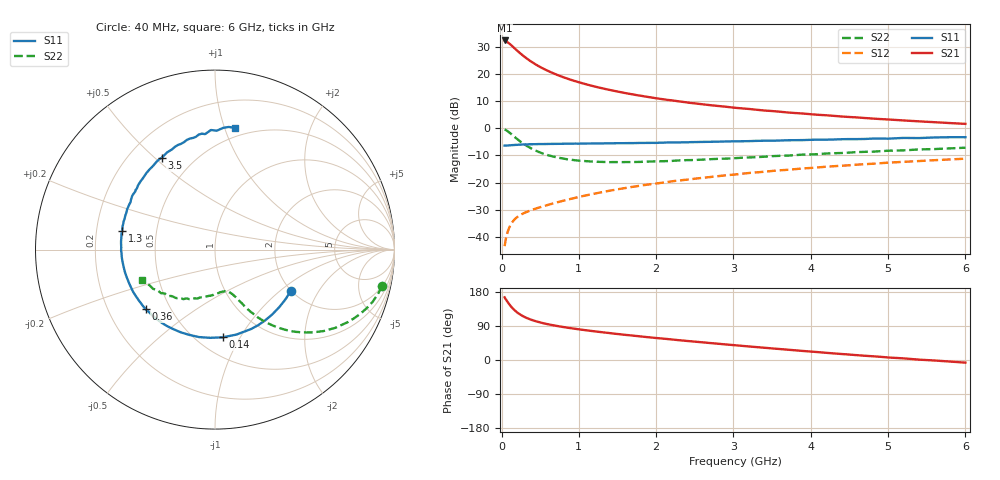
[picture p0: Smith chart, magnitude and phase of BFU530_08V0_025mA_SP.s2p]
! Filename:  P:\Prog\Test\Noise\ATS_data\Testdata_Net\03 Spar\BFU530_APG2013_40_A05_08p0V_025mA_SP_CM01_D.s2p
! Date/Time: Fri 26/Apr/2013 13:03:13
! BFU530_APG2013_40_A05_08p0V_1to25mA_SP_CM01_Bias8_R.s2p
! MDIF S-parameter v. bias file
! BFU530_APG2013_40_A05_08p0V_1to25mA_SP_CM01
! Date/time Wed Apr 24 16:58:28 2013
! VAR V_out= 7.1810
! VAR I_out= 25.0000
! VAR V_in= 0.8207
! VAR I_in= 0.2699
! Device data file deembeded for feedlines and parallel
! Original file: \03 Spar\BFU530_APG2013_40_A05_08p0V_025mA_SP_CM01_R.s2p
! Feed-files: PR047V01_250413_Feed1.s2p, PR047V01_250413_Feed2.s2p
! Parallel-file: PR047V01_250413_Par.s2p
# MHz S MA R 50
!  Freq-MHz  S11-mag  S11-arg  S21-mag  S21-arg  S12-mag  S12-arg  S22-mag  S22-arg
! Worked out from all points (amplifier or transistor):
!   98 points, 40 MHz to 6 GHz, reference 50 ohm
!   highest |S21| = 32.5 dB at 40 MHz (marker M1)
!   |S21| within 3 dB of that: start of sweep to 173.1 MHz
!   unconditionally stable (mu >= 1): 1.194 GHz to 3.436 GHz
!   at 300 MHz: K = 0.52, MSG = 28.8 dB, |S12| = -31.2 dB
!   at 1.6 GHz: K = 1.04, MAG = 16.3 dB, |S12| = -22.1 dB
!   at 6 GHz: K = 0.86, MSG = 6.4 dB, |S12| = -11.2 dB
!   S11 on the Smith chart (normalised r, x): 40 MHz: 2.00, -1.19; 140 MHz: 0.66, -0.85; 360 MHz: 0.36, -0.33; 1.3 GHz: 0.31, +0.09; 3.5 GHz: 0.33, +0.53; 6 GHz: 0.42, +1.08
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40  0.4813 -28.4  42.16 165.4  0.006663 79.8  0.9537 -12.3
50  0.4805 -35.3  41.71 161.6  0.008114 77.7  0.9405 -15.3
90  0.4849 -60.1  37.92 149.8  0.01349 69.5  0.8646 -26.2
120  0.4883 -75.9  35.01 141.8  0.01675 64.6  0.7991 -33.1
140  0.4906 -85.0  33.01 137.2  0.01855 62.0  0.756 -36.9
180  0.4954 -100.3  29.23 129.4  0.02158 58.1  0.676 -43.1
200  0.4962 -106.6  27.53 126.0  0.02279 56.6  0.6399 -45.7
240  0.5002 -117.4  24.55 120.2  0.02491 54.7  0.5769 -49.9
300  0.5052 -129.9  20.92 113.4  0.02759 53.2  0.5024 -54.5
360  0.5095 -139.3  18.1 108.1  0.02992 52.7  0.4461 -57.8
460  0.5119 -150.8  14.68 101.4  0.03356 53.3  0.379 -61.3
600  0.5152 -162.0  11.57 94.4  0.03859 54.9  0.3205 -64.3
800  0.5198 -173.0  8.821 87.0  0.04609 57.2  0.2766 -67.7
1050  0.5243 176.5  6.795 79.6  0.05601 59.1  0.251 -71.5
1300  0.5277 168.5  5.519 73.3  0.06634 60.0  0.2403 -75.4
1600  0.5335 159.9  4.495 66.4  0.07896 60.0  0.2387 -80.7
2050  0.5433 149.7  3.516 57.1  0.0979 59.0  0.247 -89.2
3100  0.5787 127.4  2.348 37.6  0.1446 54.0  0.2863 -109.0
3500  0.5914 120.2  2.091 30.6  0.1635 51.2  0.307 -115.6
4100  0.6186 109.3  1.781 20.7  0.1904 46.7  0.3345 -126.7
5200  0.6668 91.9  1.403 4.3  0.2409 37.4  0.3926 -145.0
6000  0.6871 80.7  1.212 -7.0  0.2754 29.8  0.4396 -157.6
